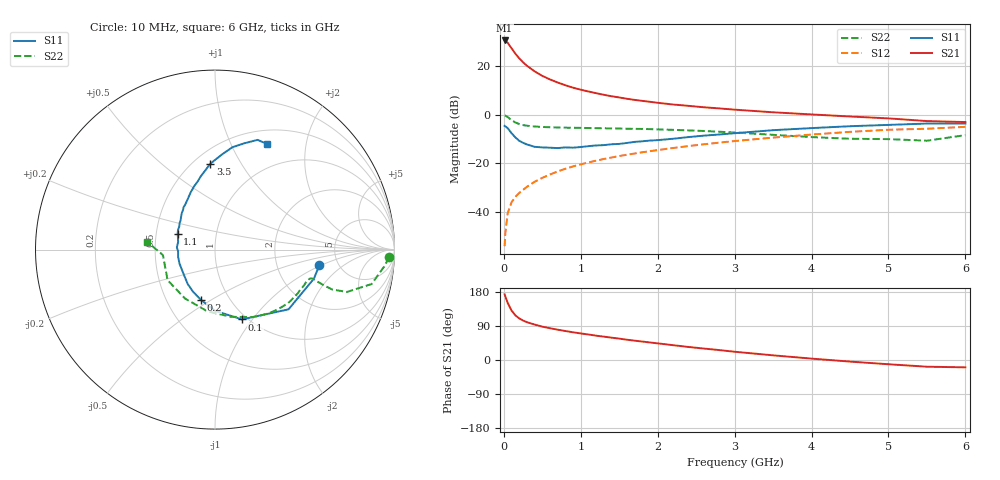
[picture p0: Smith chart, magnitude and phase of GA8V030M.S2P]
! Infineon Technologies  Discrete & RF Semiconductors
! BF775
! Si NPN RF Bipolar Junction Transistor in SOT23
! VCE = 8 V  IC = 30 mA
! Common Emitter S-Parameters:  May  1996
# GHz  S  MA  R  50
!  f  S11  S21  S12  S22
! GHz  MAG  ANG  MAG  ANG  MAG  ANG  MAG  ANG
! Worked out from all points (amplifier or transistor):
!   36 points, 10 MHz to 6 GHz, reference 50 ohm
!   highest |S21| = 30.4 dB at 10 MHz (marker M1)
!   |S21| within 3 dB of that: start of sweep to 95.84 MHz
!   unconditionally stable (mu >= 1): 326.6 MHz to 2.618 GHz
!   at 250 MHz: K = 0.93, MSG = 26.2 dB, |S12| = -30.9 dB
!   at 1.4 GHz: K = 1.12, MAG = 10.5 dB, |S12| = -17.6 dB
!   at 6 GHz: K = 0.93, MSG = 1.0 dB, |S12| = -5.0 dB
!   S11 on the Smith chart (normalised r, x): 10 MHz: 3.58, -0.94; 100 MHz: 0.95, -0.89; 200 MHz: 0.74, -0.45; 1.1 GHz: 0.65, +0.12; 3.5 GHz: 0.60, +0.75; 6 GHz: 0.67, +1.39
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0.01  0.5876 -8.4  33.26 173.4  0.002 85.4  0.9692 -2.5
0.02  0.5747 -16.3  32.7 167.2  0.0038 81.5  0.9505 -5.4
0.05  0.5278 -39.1  29.78 150.6  0.0095 76.1  0.8934 -12.4
0.1  0.4168 -68.9  23.05 130.7  0.0159 68.7  0.7721 -17.8
0.15  0.3409 -89.9  17.81 117.7  0.0205 65.8  0.689 -18.8
0.2  0.2905 -105.8  14.31 109.8  0.0247 67.8  0.6413 -18.2
0.25  0.264 -117.8  11.85 104.1  0.0286 67.7  0.6106 -17.6
0.3  0.2443 -128.6  10.08 99.8  0.033 69.6  0.5918 -17.2
0.4  0.2187 -145.1  7.727 93.5  0.0419 71.4  0.571 -16.6
0.5  0.2125 -158.5  6.239 88.0  0.0505 72.0  0.558 -16.6
0.6  0.2095 -168.7  5.273 83.9  0.0591 72.7  0.5507 -17.2
0.7  0.2058 -177.4  4.56 80.0  0.0683 73.1  0.5455 -18.1
0.8  0.2126 176.5  4.006 76.5  0.0775 72.4  0.5403 -19.1
0.9  0.2099 168.1  3.571 73.1  0.0866 72.3  0.5375 -20.2
1.1  0.2255 157.4  2.983 67.3  0.1045 71.5  0.5317 -23.1
1.3  0.2367 147.4  2.552 61.7  0.1229 70.1  0.5243 -25.8
1.6  0.2624 136.1  2.116 53.5  0.1505 67.7  0.5137 -30.8
2.2  0.3199 118.3  1.613 39.1  0.207 62.7  0.4874 -41.9
3.5  0.4795 93.1  1.117 12.3  0.3377 48.4  0.385 -76.7
4.5  0.5783 80.4  0.916 -4.2  0.4432 34.9  0.3198 -121.4
5.5  0.6558 68.8  0.738 -17.7  0.5137 18.2  0.2917 -174.0
6  0.6561 63.6  0.704 -19.4  0.5616 13.6  0.3793 173.5
